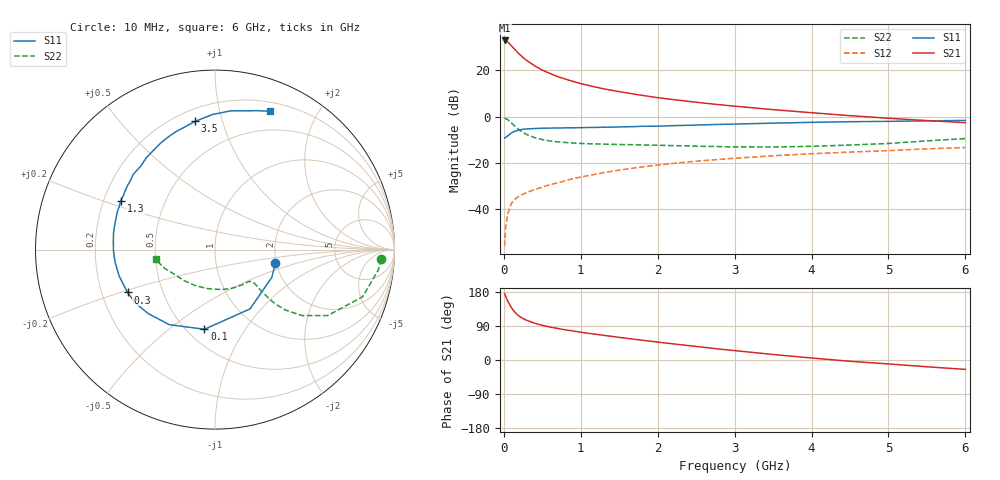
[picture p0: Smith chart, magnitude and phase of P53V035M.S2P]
! SIEMENS Small Signal Semiconductors
! BFP183
! Si NPN RF Bipolar Junction Transistor in SOT143
! VCE = 3 V  IC = 35 mA
! Common Emitter S-Parameters:  March  1996
# GHz  S  MA  R  50
!  f  S11  S21  S12  S22
! GHz  MAG  ANG  MAG  ANG  MAG  ANG  MAG  ANG
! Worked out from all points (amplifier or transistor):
!   36 points, 10 MHz to 6 GHz, reference 50 ohm
!   highest |S21| = 32.9 dB at 10 MHz (marker M1)
!   |S21| within 3 dB of that: start of sweep to 118.4 MHz
!   unconditionally stable (mu >= 1): 528.6 MHz to 5.74 GHz
!   at 250 MHz: K = 0.67, MSG = 29.5 dB, |S12| = -33.5 dB
!   at 1.4 GHz: K = 1.22, MAG = 14.7 dB, |S12| = -23.6 dB
!   at 6 GHz: K = 0.97, MSG = 5.4 dB, |S12| = -13.3 dB
!   S11 on the Smith chart (normalised r, x): 10 MHz: 1.98, -0.34; 100 MHz: 0.61, -0.67; 300 MHz: 0.31, -0.21; 1.3 GHz: 0.27, +0.23; 3.5 GHz: 0.27, +0.82; 6 GHz: 0.29, +1.44
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0.01  0.345 -12.6  44.1 174.9  0.0016 75.9  0.9272 -3.3
0.02  0.3524 -26.0  43.84 170.2  0.0037 82.1  0.9166 -7.2
0.05  0.3838 -59.4  41.09 155.8  0.008 71.9  0.8636 -17.7
0.1  0.4479 -97.6  33.7 137.4  0.0135 59.1  0.728 -30.3
0.15  0.4894 -121.3  27.39 124.6  0.0169 54.6  0.6081 -37.2
0.2  0.5152 -136.1  22.49 115.6  0.0194 52.3  0.5184 -40.6
0.25  0.5339 -146.2  18.84 109.3  0.0211 51.8  0.4555 -42.0
0.3  0.5428 -153.9  16.2 104.5  0.0232 51.3  0.4092 -42.2
0.4  0.5542 -164.7  12.53 97.0  0.0266 53.5  0.3531 -41.9
0.5  0.5614 -173.1  10.1 91.5  0.0301 54.5  0.3197 -41.3
0.6  0.5659 -179.2  8.546 87.0  0.0341 56.6  0.2991 -40.7
0.7  0.5681 175.5  7.311 83.2  0.0372 57.1  0.2855 -40.6
0.8  0.5726 171.0  6.464 79.6  0.0414 58.3  0.2768 -40.7
1.1  0.5835 159.1  4.72 70.4  0.0535 58.8  0.2603 -43.1
1.3  0.5916 152.5  3.975 65.0  0.062 58.3  0.255 -45.9
1.7  0.6095 140.2  3.046 54.6  0.0782 56.3  0.2473 -52.8
2.2  0.6391 126.8  2.338 42.5  0.0977 52.0  0.2368 -63.7
2.8  0.6796 112.5  1.813 28.8  0.1195 46.3  0.2259 -79.9
3.5  0.723 98.8  1.415 14.5  0.1429 39.8  0.2213 -101.7
4.5  0.7777 83.6  1.05 -3.4  0.1718 30.3  0.2439 -134.9
5.5  0.8102 72.8  0.823 -17.9  0.2022 21.9  0.3004 -159.9
6  0.8297 68.2  0.741 -24.7  0.2151 17.1  0.3359 -170.7
